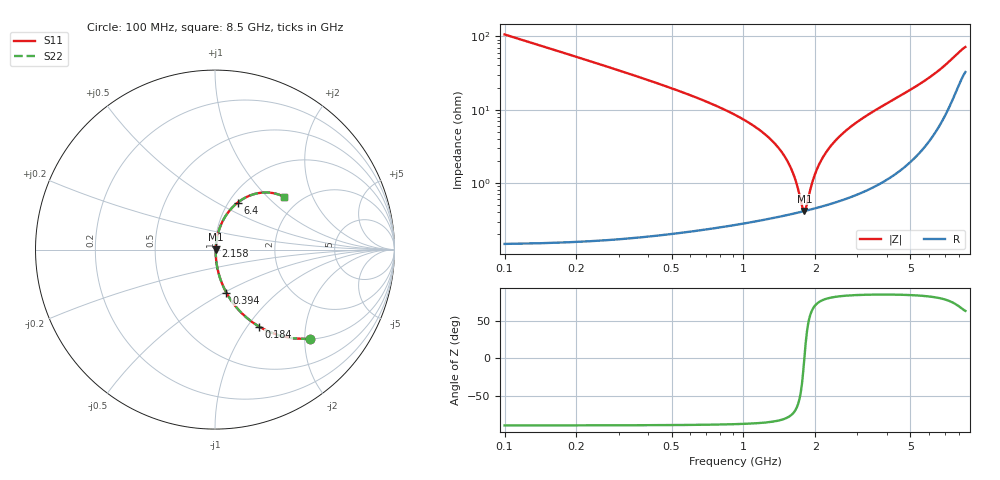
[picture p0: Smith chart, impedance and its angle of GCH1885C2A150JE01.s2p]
!Murata Part Number: GCH1885C2A150JE01
!These Parameters are Measured in Series Mode Connection
!Data Generated on Mar 13, 2026
!  o--ll--o
!Port1  Port2
!  o------o
!Operation Temp=25[degC], DC Bias Voltage=0[V]
!Freq. Start=100[MHz] Stop=9[GHz] 401[Steps]
# Hz S RI R 50
!Freq.(Hz) S11(Real) S11(Imag) S21(Real) S21(Imag) S12(Real) S12(Imag) S22(Real) S22(Imag)
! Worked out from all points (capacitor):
!   401 points, 100 MHz to 8.5 GHz, reference 50 ohm
!   read as one part in series: C = 15 pF near 142 MHz
!   lowest |Z| = 416 mohm at 1.801 GHz (marker M1)
!   series resonance near 1.8 GHz, so ESL is about 520 pH
!   S11 on the Smith chart (normalised r, x): 100 MHz: 1.00, -2.12; 184 MHz: 1.00, -1.14; 394 MHz: 1.00, -0.51; 2.158 GHz: 1.01, +0.04; 6.4 GHz: 1.10, +0.63; 8.5 GHz: 1.65, +1.27
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1e8  0.528 -0.4985  0.472 0.4985  0.472 0.4985  0.528 -0.4985
1.84e8  0.2461 -0.4294  0.7539 0.4294  0.7539 0.4294  0.2461 -0.4294
2.68e8  0.1313 -0.3356  0.8687 0.3356  0.8687 0.3356  0.1313 -0.3356
3.94e8  0.0631 -0.2396  0.9369 0.2396  0.9369 0.2396  0.0631 -0.2396
7.09e8  0.018 -0.1239  0.982 0.1239  0.982 0.1239  0.018 -0.1239
1.234e9  0.00525 -0.0455  0.9947 0.0455  0.9947 0.0455  0.00525 -0.0455
1.507e9  0.00408 -0.0211  0.9959 0.0211  0.9959 0.0211  0.00408 -0.0211
1.633e9  0.00398 -0.0116  0.996 0.0116  0.996 0.0116  0.00398 -0.0116
1.759e9  0.00407 -0.00272  0.9959 0.00272  0.9959 0.00272  0.00407 -0.00272
1.801e9  0.00414 9.5e-05  0.9959 -9.5e-05  0.9959 -9.5e-05  0.00414 9.5e-05
1.843e9  0.00423 0.00285  0.9958 -0.00285  0.9958 -0.00285  0.00423 0.00285
1.927e9  0.00445 0.00821  0.9956 -0.00821  0.9956 -0.00821  0.00445 0.00821
1.99e9  0.00465 0.0121  0.9954 -0.0121  0.9954 -0.0121  0.00465 0.0121
2.158e9  0.00532 0.0221  0.9947 -0.0221  0.9947 -0.0221  0.00532 0.0221
2.473e9  0.0071 0.0395  0.9929 -0.0395  0.9929 -0.0395  0.0071 0.0395
2.914e9  0.0106 0.0624  0.9894 -0.0624  0.9894 -0.0624  0.0106 0.0624
3.502e9  0.0173 0.092  0.9827 -0.092  0.9827 -0.092  0.0173 0.092
4.3e9  0.0313 0.1335  0.9687 -0.1335  0.9687 -0.1335  0.0313 0.1335
5.707e9  0.0806 0.2169  0.9194 -0.2169  0.9194 -0.2169  0.0806 0.2169
6.4e9  0.1268 0.2622  0.8732 -0.2622  0.8732 -0.2622  0.1268 0.2622
7.114e9  0.2005 0.3035  0.7995 -0.3035  0.7995 -0.3035  0.2005 0.3035
8.5e9  0.387 0.2945  0.613 -0.2945  0.613 -0.2945  0.387 0.2945
